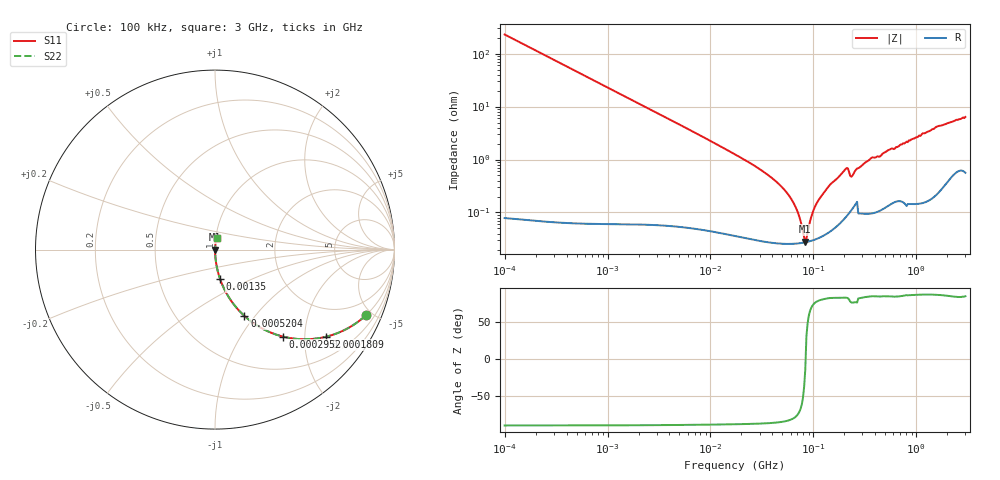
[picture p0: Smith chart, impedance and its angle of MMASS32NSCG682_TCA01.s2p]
! MMASS32NSCG682_TCA01  S-PARAMETER MODEL  ( Standard Model )
! Model Generated by TAIYO YUDEN Corporation (https://www.yuden.co.jp/en/)
! Version 1.0
! TAIYO YUDEN Control No. 250312
! Copyright(c) 2025 TAIYO YUDEN CO.,LTD. All Rights Reserved.
! Product Description (link to TY-COMPAS)
! https://ds.yuden.co.jp/TYCOMPAS/or/detail?pn=MMASS32NSCG682JTCA01&u=M
! Products Name : Multilayer Ceramic Capacitors
! Characteristics :
!  Capacitance : 6800 [pF] , Rated Voltage : 630 [V] , TCC : CG / C0G
!  Case Size : 3.2 x 2.5 / 0.126 x 0.098 [mm/inch] , Thickness : 1.9 / 0.075 [mm/inch]
!  (Conditions: Temperature = 25 [degC] , DC Bias Voltage = 0 [V])
! External Node Assignments :
!  1  o---| |---o  2
! GND o---------o GND
! Frequency Range : 0.1MHz  -  3000MHz  [ 401 STEP ]
# MHZ S RI R 50
! Freq[MHz].  S11 Real  S11 Imag  S21 Real  S21 Imag  S12 Real  S12 Imag  S22 Real  S22 Imag
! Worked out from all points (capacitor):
!   401 points, 100 kHz to 3 GHz, reference 50 ohm
!   read as one part in series: C = 6.92 nF near 105.3 kHz
!   lowest |Z| = 28.3 mohm at 83.43 MHz (marker M1)
!   series resonance near 84.09 MHz, so ESL is about 520 pH
!   S11 on the Smith chart (normalised r, x): 100 kHz: 1.00, -4.60; 180.9 kHz: 1.00, -2.54; 295.2 kHz: 1.00, -1.56; 520.4 kHz: 1.00, -0.88; 1.35 MHz: 1.00, -0.34; 3 GHz: 1.01, +0.13
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0.1  0.8411 -0.3654  0.1589 0.3654  0.1589 0.3654  0.8411 -0.3654
0.180898  0.6178 -0.4856  0.3822 0.4856  0.3822 0.4856  0.6178 -0.4856
0.295187  0.3779 -0.4844  0.6221 0.4844  0.6221 0.4844  0.3779 -0.4844
0.520403  0.1638 -0.3694  0.8362 0.3694  0.8362 0.3694  0.1638 -0.3694
0.562235  0.1438 -0.3501  0.8562 0.3501  0.8562 0.3501  0.1438 -0.3501
1.350433  0.0287 -0.1652  0.9713 0.1652  0.9713 0.1652  0.0287 -0.1652
3.161081  0.00581 -0.0722  0.9942 0.0722  0.9942 0.0722  0.00581 -0.0722
17.7727  0.000503 -0.0122  0.9995 0.0122  0.9995 0.0122  0.000503 -0.0122
34.73492  0.000306 -0.00542  0.9997 0.00542  0.9997 0.00542  0.000306 -0.00542
52.46276  0.000263 -0.00266  0.9997 0.00266  0.9997 0.00266  0.000263 -0.00266
67.88584  0.00026 -0.00119  0.9997 0.00119  0.9997 0.00119  0.00026 -0.00119
83.42988  0.000273 -7.16e-05  0.9997 7.16e-05  0.9997 7.16e-05  0.000273 -7.16e-05
87.84301  0.00028 0.000309  0.9997 -0.000309  0.9997 -0.000309  0.00028 0.000309
97.38194  0.000296 0.000891  0.9997 -0.000891  0.9997 -0.000891  0.000296 0.000891
107.9567  0.00032 0.00147  0.9997 -0.00147  0.9997 -0.00147  0.00032 0.00147
122.8043  0.000361 0.00216  0.9996 -0.00216  0.9996 -0.00216  0.000361 0.00216
200.3904  0.0008 0.00622  0.9992 -0.00622  0.9992 -0.00622  0.0008 0.00622
240.0085  0.0012 0.00484  0.9988 -0.00484  0.9988 -0.00484  0.0012 0.00484
353.2796  0.00105 0.01  0.999 -0.01  0.999 -0.01  0.00105 0.01
547.5153  0.00161 0.0152  0.9984 -0.0152  0.9984 -0.0152  0.00161 0.0152
1616.196  0.00406 0.0422  0.9959 -0.0422  0.9959 -0.0422  0.00406 0.0422
3000  0.00952 0.0624  0.9905 -0.0624  0.9905 -0.0624  0.00952 0.0624
